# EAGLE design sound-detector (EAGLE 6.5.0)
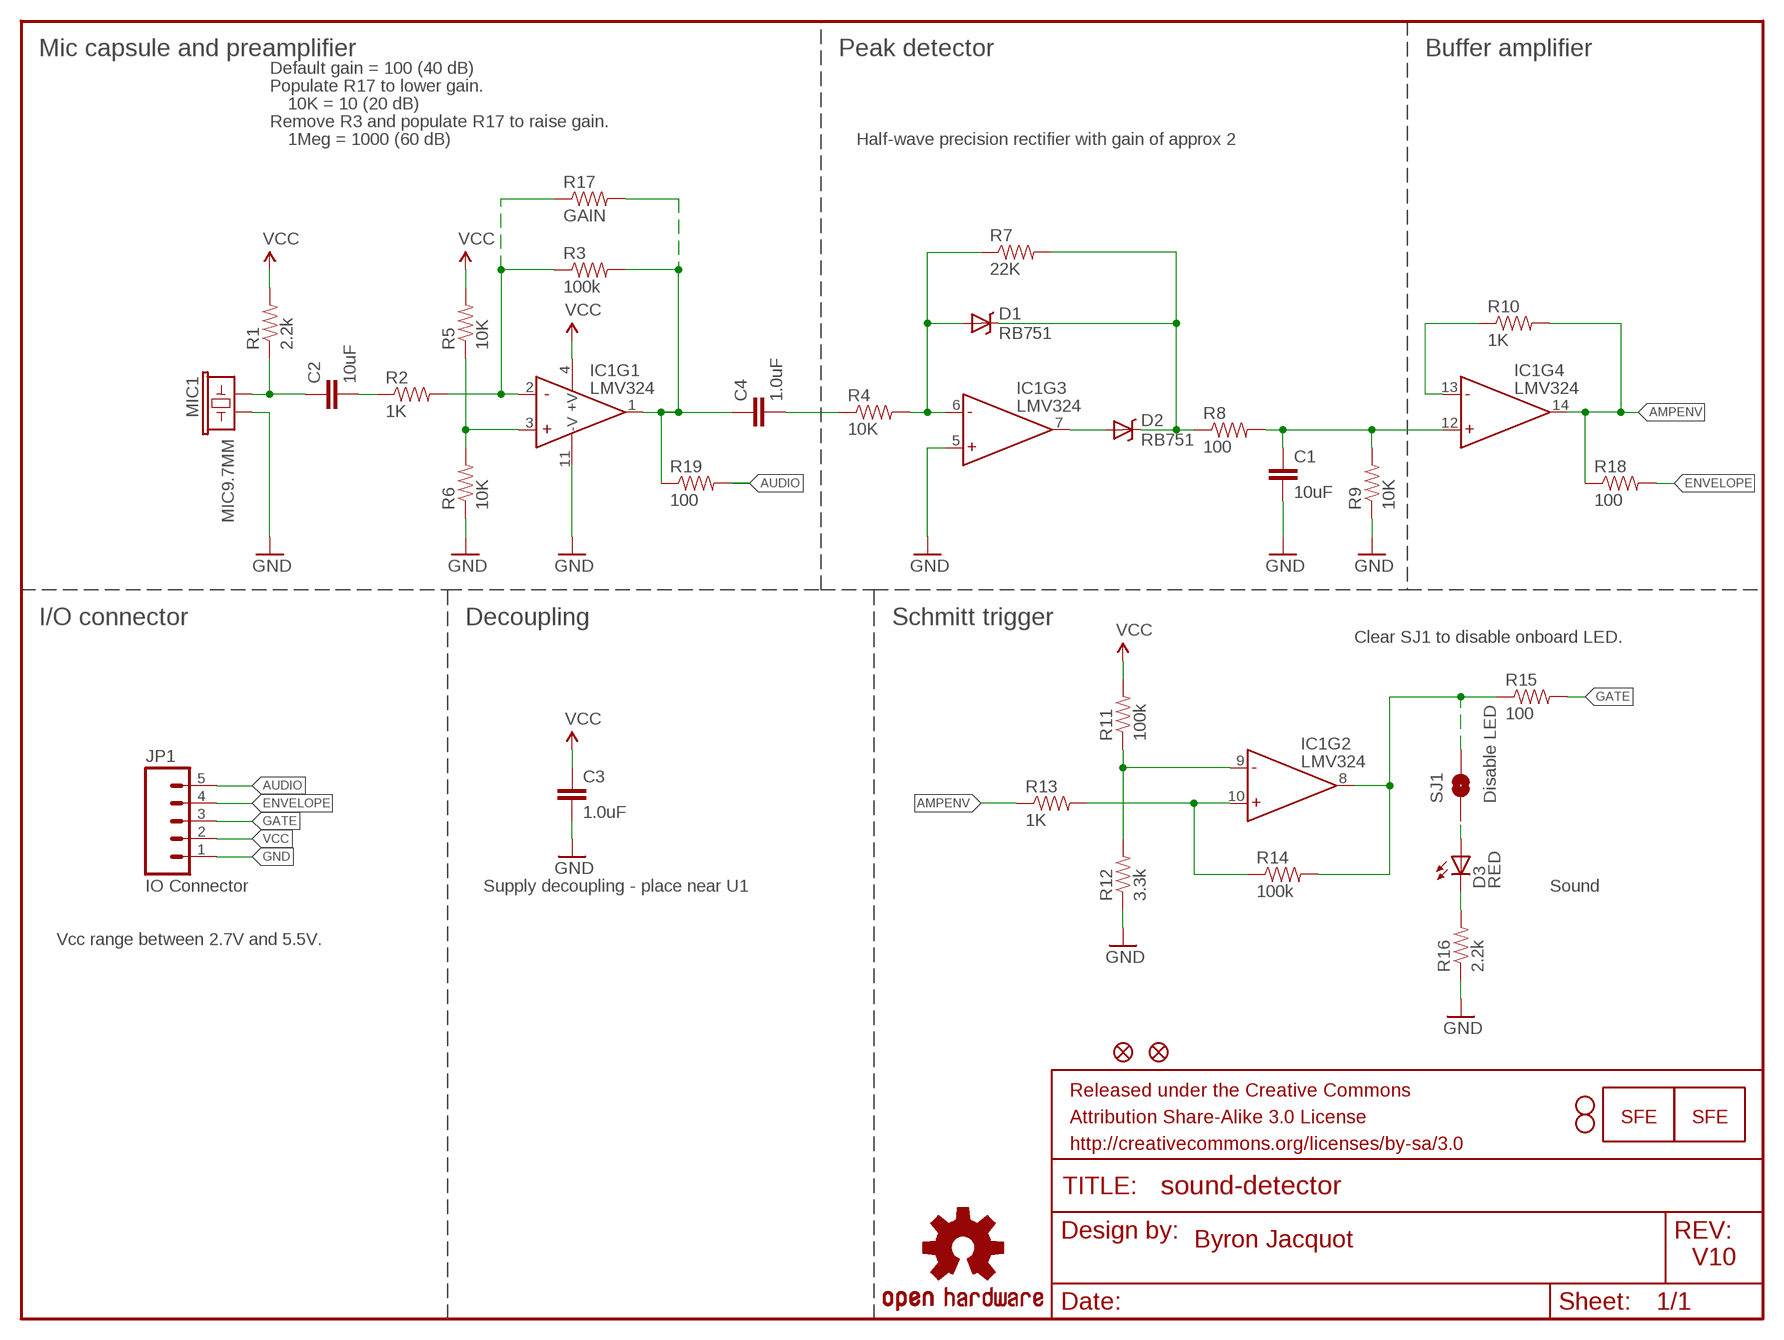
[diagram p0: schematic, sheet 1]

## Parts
C1  10uF  10UF-6.3V-20%(1206)  [1206]
C2  10uF  10UF-6.3V-20%(1206)  [1206]
C3  1.0uF  1.0UF-16V-10%(0603)  [0603-CAP]
C4  1.0uF  1.0UF-16V-10%(0603)  [0603-CAP]
D1  RB751  [SOD-523]
D2  RB751  [SOD-523]
D3  RED  LED-RED0603  [LED-0603]
FID1  FIDUCIALUFIDUCIAL  [MICRO-FIDUCIAL]
FID2  FIDUCIALUFIDUCIAL  [MICRO-FIDUCIAL]
FRAME1  FRAME-LETTER  [CREATIVE_COMMONS]
IC1  LMV324  [SO014]
JP1  IO Connector  M05PTH  [1X05]
LOGO1  OSHW-LOGOM  [OSHW-LOGO-M]
LOGO2  LOGO-SFENW2  [SFE-NEW-WEB]
LOGO3  LOGO-SFESK  [SFE-LOGO-FLAME]
MIC1  MIC9.7MM  [MIC-9.7MM]
R1  2.2k  2.2KOHM1/10W1%(0603)  [0603-RES]
R2  1K  1KOHM1/10W1%(0603)  [0603-RES]
R3  100k  100KOHM1/10W1%(0603)  [0603-RES]
R4  10K  10KOHM1/10W1%(0603)0603  [0603-RES]
R5  10K  10KOHM1/10W1%(0603)0603  [0603-RES]
R6  10K  10KOHM1/10W1%(0603)0603  [0603-RES]
R7  22K  22KOHM1/10W1%(0603)  [0603-RES]
R8  100  100OHM1/10W1%(0603)  [0603-RES]
R9  10K  10KOHM1/10W1%(0603)0603  [0603-RES]
R10  1K  1KOHM1/10W1%(0603)  [0603-RES]
R11  100k  100KOHM1/10W1%(0603)  [0603-RES]
R12  3.3k  3.3KOHM1/10W1%(0603)  [0603-RES]
R13  1K  1KOHM1/10W1%(0603)  [0603-RES]
R14  100k  100KOHM1/10W1%(0603)  [0603-RES]
R15  100  100OHM1/10W1%(0603)  [0603-RES]
R16  2.2k  2.2KOHM1/10W1%(0603)  [0603-RES]
R17  GAIN  RESISTORPTH-1/4W-VERT-KIT  [AXIAL-0.1EZ]
R18  100  100OHM1/10W1%(0603)  [0603-RES]
R19  100  100OHM1/10W1%(0603)  [0603-RES]
SJ1  Disable LED  SOLDERJUMPERNC  [SJ_2S]
STANDOFF1  STAND-OFF  [STAND-OFF]
STANDOFF2  STAND-OFF  [STAND-OFF]

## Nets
AMPENV: IC1.14(OUT) R10.2 R13.1 R18.1
AUDIO: JP1.5 R19.2
ENVELOPE: JP1.4 R18.2
GATE: JP1.3 R15.2
GND: C1.2 C3.2 IC1.5(+IN) IC1.11(-V) JP1.1 MIC1.2 R6.1 R9.1 R12.1 R16.1
N$: C4.1 IC1.1(OUT) R3.2 R17.P$2 R19.1
N$1: C2.1 MIC1.1 R1.1
N$2: IC1.3(+IN) R5.1 R6.2
N$3: D3.C R16.2
N$4: IC1.2(-IN) R2.2 R3.1 R17.P$1
N$5: C2.2 R2.1
N$6: C4.2 R4.1
N$7: D1.A IC1.6(-IN) R4.2 R7.1
N$8: D2.A IC1.7(OUT)
N$9: D1.C D2.C R7.2 R8.1
N$10: C1.1 IC1.12(+IN) R8.2 R9.2
N$11: IC1.13(-IN) R10.1
N$12: D3.A SJ1.1
N$15: IC1.9(-IN) R11.1 R12.2
N$16: IC1.10(+IN) R13.2 R14.1
N$17: IC1.8(OUT) R14.2 R15.1 SJ1.2
VCC: C3.1 IC1.4(+V) JP1.2 R1.2 R5.2 R11.2

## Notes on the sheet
- Mic capsule and preamplifier | Peak detector | Buffer amplifier
- Default gain = 100 (40 dB)
- Populate R17 to lower gain.
- 10K = 10 (20 dB)
- Remove R3 and populate R17 to raise gain.
- 1Meg = 1000 (60 dB) | Half-wave precision rectifier with gain of approx 2
- I/O connector | Decoupling | Schmitt trigger
- Clear SJ1 to disable onboard LED.
- Supply decoupling - place near U1 | Sound
- Vcc range between 2.7V and 5.5V.
- Byron Jacquot
- V10

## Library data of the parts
C1 C2 = SparkFun-Capacitors:10UF-6.3V-20%(1206): Ceramic; PROD_ID: CAP-10057
C3 C4 = SparkFun-Capacitors:1.0UF-16V-10%(0603): CAP-00868; PROD_ID: CAP-00868
D1 D2 = SparkFun-DiscreteSemi:RB751: 40V 120mA SOD-523 Schottky; PROD_ID: DIO-11018
D3 = SparkFun-LED:LED-RED: Assorted Red LEDs; PROD_ID: DIO-00819
FID1 FID2 = SparkFun-Aesthetics:FIDUCIAL: Fiducial Alignment Points
FRAME1 = SparkFun-Aesthetics:FRAME-LETTER: Schematic Frame
IC1 = SparkFun-AnalogIC:LMV324: Jellybean quad op-amp; PROD_ID: IC-08227
JP1 = SparkFun-Connectors:M05: Header 5 Standard 5-pin 0.1" header. Use with straight break away headers (SKU : PRT-00116), right angle break away headers (PRT-00553), swiss pins (PRT-00743), machine pins (PRT-00117), and female headers (PRT-00115). Molex polarized connector foot print use with SKU : PRT-08230 with associated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
LOGO1 = SparkFun-Aesthetics:OSHW-LOGO: Open Source Hardware Logo This logo indicates the piece of hardware it is found on incorporates a OSHW license and/or adheres to the definition of open source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
LOGO2 LOGO3 = SparkFun-Aesthetics:LOGO-SFE: Spark Fun Electronics PCB Logo
MIC1 = SparkFun-Sensors:MIC: Omni-directional electret microphone. 9.7mm standard diameter.; PROD_ID: COMP-08856
R1 R16 = SparkFun-Resistors:2.2KOHM1/10W1%(0603): RES-08272; PROD_ID: RES-08272
R2 R10 R13 = SparkFun-Resistors:1KOHM1/10W1%(0603): RES-07856; PROD_ID: RES-07856
R3 R11 R14 = SparkFun-Resistors:100KOHM1/10W1%(0603): RES-07828; PROD_ID: RES-07828
R4-R6 R9 = SparkFun-Resistors:10KOHM1/10W1%(0603): RES-00824; PROD_ID: RES-00824
R7 = SparkFun-Resistors:22KOHM1/10W1%(0603): RES-07853; PROD_ID: RES-07853
R8 R15 R18 R19 = SparkFun-Resistors:100OHM1/10W1%(0603): RES-07863; PROD_ID: RES-07863
R12 = SparkFun-Resistors:3.3KOHM1/10W1%(0603): RES-07851; PROD_ID: RES-07851
R17 = SparkFun-Resistors:RESISTOR: Resistor
SJ1 = SparkFun-Passives:SOLDERJUMPER: Solder Jumper
STANDOFF1 STANDOFF2 = SparkFun-Electromechanical:STAND-OFF: #4 Stand Off

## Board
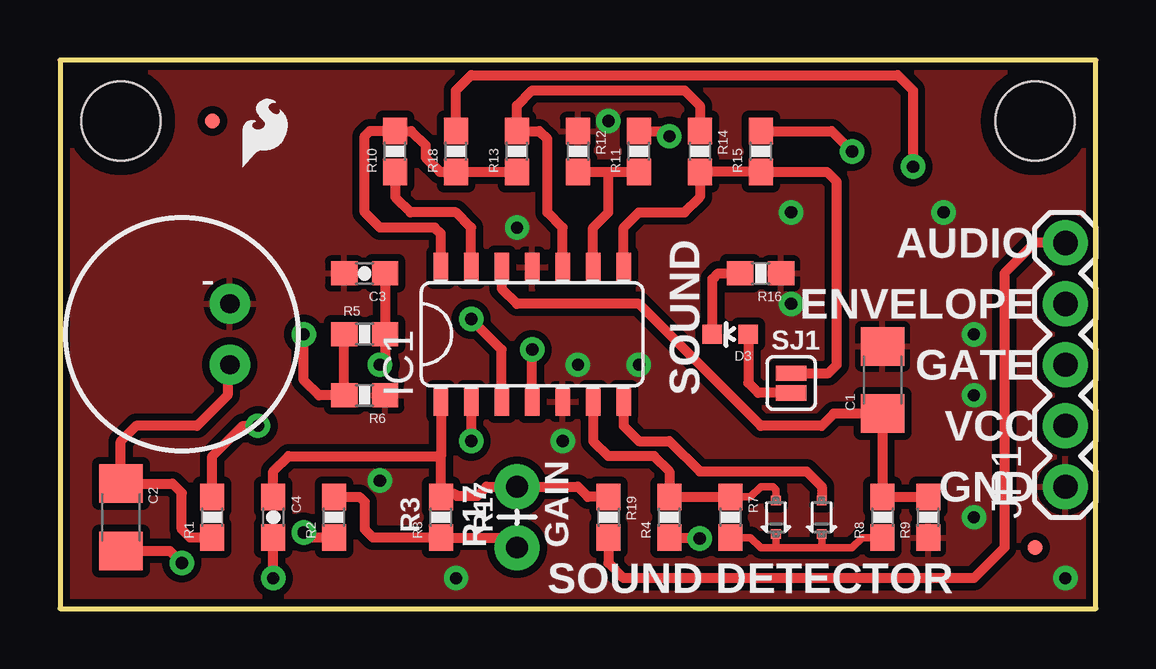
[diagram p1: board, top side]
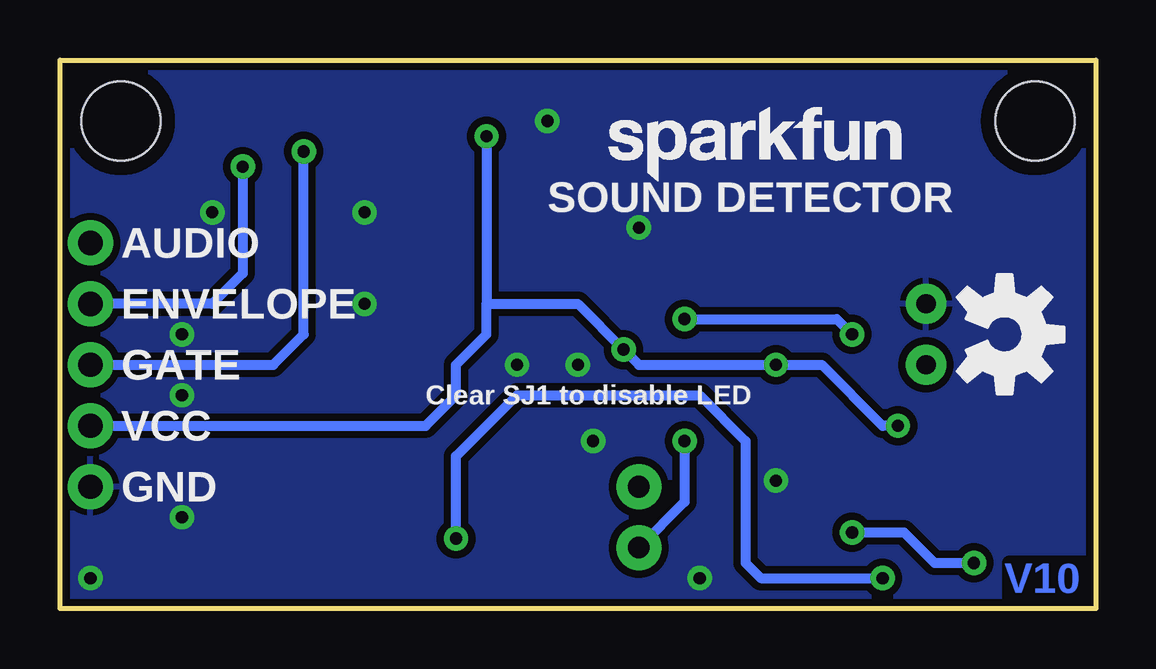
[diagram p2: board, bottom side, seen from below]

Size 43.18 x 22.86 mm. Coordinates in mm from the lower left corner, seen from the top.
Outline: 0,0 43.18,0 43.18,22.86 0,22.86 0,0
Copper layers (1*16): Top 0.035mm / dielectric 1.5mm / Bottom 0.035mm
Design rules "SparkFun-2-layer *": minimum track width 7mil, minimum drill 15mil, track to track 8mil, track to pad 8mil, pad to pad 8mil, via to via 8mil, smd to smd 8mil, copper to edge 8mil, drill to drill 8mil, minimum pad ring 12mil, minimum via ring 10mil, stop-mask expansion 4mil, vias tented up to drill 20mil, thermal gap 10mil

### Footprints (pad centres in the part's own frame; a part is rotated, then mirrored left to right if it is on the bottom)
1206 = smd 1.6 x 1.8: 1 -1.4,0; 2 1.4,0
0603-CAP = smd 1.1 x 1: 1 -0.85,0; 2 0.85,0
SOD-523 = smd 0.4 x 0.4: A -0.7,0; C 0.7,0
LED-0603 = smd 0.8 x 0.8: A 0,-0.75; C 0,0.75
MICRO-FIDUCIAL = smd 0.635 x 0.635: 1 0,0
SO014 = smd 0.6 x 1.2: 1 -3.175,-2.8; 2 -1.905,-2.8; 3 -0.635,-2.8; 4 0.635,-2.8; 5 1.905,-2.8; 6 3.175,-2.8; 7 4.445,-2.8; 8 4.445,2.8; 9 3.175,2.8; 10 1.905,2.8; 11 0.635,2.8; 12 -0.635,2.8; 13 -1.905,2.8; 14 -3.175,2.8
1X05 = drill 1.016 pad 1.88: 1 0,0; 2 2.54,0; 3 5.08,0; 4 7.62,0; 5 10.16,0
MIC-9.7MM = drill 0.8 pad 1.676: 1 -2,1.27; 2 -2,-1.27
0603-RES = smd 1.1 x 1: 1 -0.85,0; 2 0.85,0
AXIAL-0.1EZ = drill 0.9 pad 1.88: P$1 0,0; P$2 2.54,0
SJ_2S = smd 0.635 x 1.27: 1 -0.412,0; 2 0.412,0
STAND-OFF = hole 3.302: 0,0

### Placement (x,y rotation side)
C1  34.29,9.53 90 top
C2  2.54,3.81 270 top
C3  12.7,13.97 180 top
C4  8.89,3.81 270 top
D1  29.84,3.81 270 top
D2  31.75,3.81 270 top
D3  27.94,11.43 90 top
FID1  6.35,20.32 0 top
FID2  40.64,2.54 0 top
FRAME1  not placed on the board
IC1  19.05,11.43 0 top
JP1  41.91,5.08 90 top
LOGO1  3.81,11.43 270 bottom
LOGO2  20.32,17.78 0 bottom
LOGO3  7.62,18.41 0 top
MIC1  5.08,11.43 180 top
R1  6.35,3.81 90 top
R2  11.43,3.81 90 top
R3  15.88,3.81 90 top
R4  25.4,3.81 90 top
R5  12.7,11.43 0 top
R6  12.7,8.89 180 top
R7  27.94,3.81 270 top
R8  34.29,3.81 90 top
R9  36.2,3.81 90 top
R10  13.97,19.05 90 top
R11  24.13,19.05 90 top
R12  21.59,19.05 270 top
R13  19.05,19.05 90 top
R14  26.67,19.05 270 top
R15  29.21,19.05 90 top
R16  29.21,13.97 180 top
R17  19.05,2.54 90 top
R18  16.51,19.05 90 top
R19  22.86,3.81 270 top
SJ1  30.48,9.4 90 top
STANDOFF1  2.54,20.32 0 top
STANDOFF2  40.64,20.32 0 top

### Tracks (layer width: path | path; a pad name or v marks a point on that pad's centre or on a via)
AMPENV
  Top 0.406: R13.1 R18.1 15.84,18.2 15.24,18.8 15.24,19.3 14.64,19.9 R10.2 12.91,19.9 12.7,19.68 12.7,16.51 13.34,15.88 15.62,15.88 15.88,15.62 IC1.14
AUDIO
  Top 0.406: JP1.5 40.64,15.24 39.37,13.97 39.37,2.54 38.1,1.27 23.5,1.27 22.86,1.91 R19.2
ENVELOPE  (via drill 0.51)
  Top 0.406: R18.2 16.51,21.59 17.14,22.23 34.92,22.23 35.56,21.59 v35.56,18.41
  Bottom 0.406: v35.56,18.41 35.56,13.97 36.83,12.7 JP1.4
GATE  (via drill 0.51)
  Top 0.406: R15.2 32.17,19.9 v33.02,19.05
  Bottom 0.406: JP1.3 34.29,10.16 33.02,11.43 v33.02,19.05
GND  (via drill 0.51)
  other vias: 22.86,20.32 19.05,15.88 38.1,3.81 38.1,8.89 36.83,16.51 38.1,11.43 24.13,10.16 21.59,10.16 41.91,1.27 16.51,1.27 30.48,16.51 30.48,12.7 13.34,5.33 20.95,6.99
  pour Bottom (isolate 0.305): 0,0 0,22.86 43.18,22.86 43.18,0
  pour Top (isolate 0.305): 0,0 0,22.86 43.18,22.86 43.18,0
N$
  Top 0.406: IC1.1 15.88,6.35 | 15.88,6.35 R3.2 arc-90 16.55,4.7 17.4,4.7 17.78,5.08 R17.P$2 21.59,5.08 22.01,4.66 R19.1 | C4.1 8.89,5.71 9.53,6.35 15.88,6.35
N$1
  Top 0.406: MIC1.1 6.99,10.06 6.99,8.89 5.71,7.62 3.17,7.62 2.54,6.99 C2.1 4.7,5.21 5.08,4.83 5.08,3.3 5.42,2.96 R1.1
N$2  (via drill 0.51)
  Top 0.406: R5.1 R6.2 10.79,8.89 10.16,9.53 v10.16,11.43 | IC1.3 18.41,10.79 v17.14,12.06
  Bottom 0.406: v17.14,12.06 10.79,12.06 v10.16,11.43
N$3
  Top 0.406: D3.C 27.19,13.73 27.43,13.97 R16.2
N$4  (via drill 0.51)
  Top 0.406: R17.P$1 18.63,2.96 R3.1 13.04,2.96 12.7,3.3 12.7,4.45 12.48,4.66 R2.2 | IC1.2 v17.14,6.99
  Bottom 0.406: v17.14,6.99 17.14,4.45 R17.P$1
N$5  (via drill 0.51)
  Top 0.406: R2.1 10.38,2.96 v10.16,3.17 | C2.2 4.58,2.41 v5.08,1.91
  Bottom 0.406: v10.16,3.17 8,3.17 6.73,1.91 v5.08,1.91
N$6  (via drill 0.51)
  Top 0.406: v8.89,1.27 C4.2 | 25.36,2.96 R4.1 26.63,2.96 v26.67,2.92
  Bottom 0.406: v26.67,2.92 26.67,6.35 24.13,8.89 16.51,8.89 14.61,6.99 14.61,1.91 13.97,1.27 v8.89,1.27
N$7
  Top 0.305: D1.A 29.84,4.95 29.72,5.08 29.21,5.08 28.79,4.66 R7.1
  Top 0.406: IC1.6 22.23,6.99 22.86,6.35 24.77,6.35 25.4,5.71 R4.2 R7.1 | 28.24,4.36 R7.1 | 27.94,4.51 R7.1
N$8
  Top 0.406: IC1.7 23.5,7.62 24.13,6.99 25.4,6.99 26.67,5.71 31.11,5.71 31.75,5.08 D2.A
N$9
  Top 0.305: 29.84,2.54 29.21,2.54 28.79,2.96 R7.2 | 29.84,2.54 31.75,2.54 | 31.75,2.54 33.02,2.54 33.44,2.96 R8.1 | D1.C 29.84,2.54 | D2.C 31.75,2.54
  Top 0.406: 27.94,3.11 R7.2 | 34.29,3.11 R8.1
N$10
  Top 0.406: R9.2 R8.2 C1.1 32.26,8.12 31.75,7.62 29.21,7.62 24.13,12.7 19.05,12.7 18.41,13.34 IC1.12
N$11
  Top 0.406: R10.1 13.97,17.14 14.61,16.51 16.51,16.51 17.14,15.88 IC1.13
N$12
  Top 0.406: SJ1.1 29.11,8.99 28.69,9.41 D3.A
N$15
  Top 0.406: R12.2 22.86,18.2 | 22.86,18.2 R11.1 | IC1.9 22.23,15.88 22.86,16.51 22.86,18.2
N$16
  Top 0.406: R14.1 26.67,20.95 26.04,21.59 19.68,21.59 19.05,20.95 R13.2 19.98,19.9 20.32,19.56 20.32,16.51 20.95,15.88 IC1.10
N$17
  Top 0.406: SJ1.2 32.03,9.81 32.38,10.16 32.38,17.78 31.96,18.2 R15.1 R14.2 26.67,17.14 26.04,16.51 24.13,16.51 23.5,15.88 IC1.8
VCC  (via drill 0.51)
  Top 0.406: C3.1 R5.2 13.55,10.38 v13.34,10.16 | R1.2 6.35,6.35 7.62,7.62 v8.26,7.62 | IC1.4 v19.68,10.79 | R11.2 25.18,19.9 v25.4,19.68
  Bottom 0.406: JP1.2 27.94,7.62 26.67,8.89 26.67,10.16 25.4,11.43 25.4,12.7 | 25.4,12.7 21.59,12.7 v19.68,10.79 19.05,10.16 v13.34,10.16 11.43,10.16 8.89,7.62 v8.26,7.62 | v25.4,19.68 25.4,12.7

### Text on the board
Bottom: V10
tPlace: AUDIO | ENVELOPE | GATE | SOUND | VCC | GND | R3 | R17 | SOUND DETECTOR
bPlace: SOUND DETECTOR | AUDIO | ENVELOPE | GATE | Clear SJ1 to disable LED | VCC | GND
tDocu: Byron Jacquot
